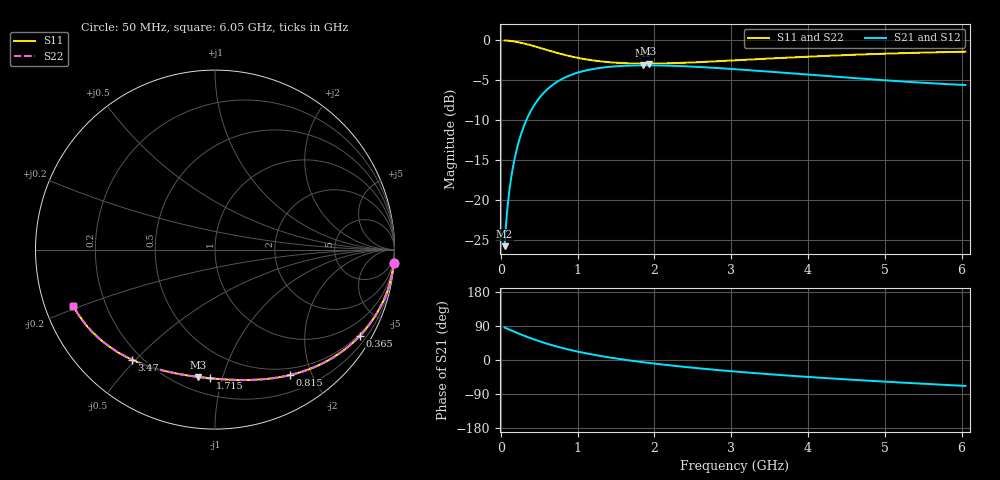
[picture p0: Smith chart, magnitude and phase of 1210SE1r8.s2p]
! AVX Thin Film Operation		Date: August 2001
! Description: Accu-P® Series, Thin Film, SMD, RF Capacitor
! Part Number: 12101J1R8ABT
! 50 MHz  -  6.05 GHz
! Serial Measurements
# mhz S db R 50
!	S11		S21		S12		S22
!	dB	Phase	dB	Phase	dB	Phase	dB	Phase
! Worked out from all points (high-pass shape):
!   401 points, 50 MHz to 6.05 GHz, reference 50 ohm
!   highest |S21| = -3.12 dB at 1.85 GHz (marker M1); lowest = -25.7 dB at 50 MHz (marker M2)
!   |S21| within 3 dB of the highest: 605.5 MHz to end of sweep
!   lowest |S11| = -2.9 dB at 1.925 GHz (marker M3), VSWR 6.03, Z = 14.3 - j41.6 ohm
!   |S11| at or under -10 dB: nowhere
!   |S22| runs from -2.9 to 0.0 dB; largest |S21 - S12| = 0
!   S11 on the Smith chart (normalised r, x): 50 MHz: 0, -26; 365 MHz: 0.44, -3.59; 815 MHz: 0.41, -1.69; 1.715 GHz: 0.31, -0.91; 3.47 GHz: 0.16, -0.49; 6.05 GHz: 0.08, -0.19
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50  -0.01 -4.4  -25.72 85.6  -25.72 85.6  -0.01 -4.4
65  -0.02 -5.8  -23.46 84.3  -23.46 84.3  -0.02 -5.8
110  -0.06 -9.7  -18.94 80.3  -18.94 80.3  -0.06 -9.7
140  -0.09 -12.3  -16.90 77.7  -16.90 77.7  -0.09 -12.3
170  -0.13 -14.9  -15.28 75.1  -15.28 75.1  -0.13 -14.9
260  -0.29 -22.4  -11.85 67.6  -11.85 67.6  -0.29 -22.4
365  -0.54 -30.7  -9.30 59.3  -9.30 59.3  -0.54 -30.7
455  -0.79 -37.3  -7.81 52.7  -7.81 52.7  -0.79 -37.3
575  -1.13 -45.3  -6.40 44.7  -6.40 44.7  -1.13 -45.3
815  -1.78 -59.0  -4.74 31.0  -4.74 31.0  -1.78 -59.0
1055  -2.28 -70.1  -3.89 19.9  -3.89 19.9  -2.28 -70.1
1355  -2.68 -81.3  -3.37 8.7  -3.37 8.7  -2.68 -81.3
1715  -2.89 -92.2  -3.14 -2.2  -3.14 -2.2  -2.89 -92.2
1850  -2.91 -95.8  -3.12 -5.8  -3.12 -5.8  -2.91 -95.8
1925  -2.91 -97.7  -3.12 -7.7  -3.12 -7.7  -2.91 -97.7
2060  -2.89 -100.9  -3.13 -10.9  -3.13 -10.9  -2.89 -100.9
2540  -2.74 -111.2  -3.30 -21.2  -3.30 -21.2  -2.74 -111.2
3050  -2.50 -120.4  -3.60 -30.4  -3.60 -30.4  -2.50 -120.4
3470  -2.29 -127.1  -3.89 -37.1  -3.89 -37.1  -2.29 -127.1
4055  -2.01 -135.4  -4.32 -45.5  -4.32 -45.5  -2.01 -135.4
5060  -1.65 -147.7  -5.03 -57.8  -5.03 -57.8  -1.65 -147.7
6050  -1.42 -158.3  -5.58 -68.4  -5.58 -68.4  -1.42 -158.3
